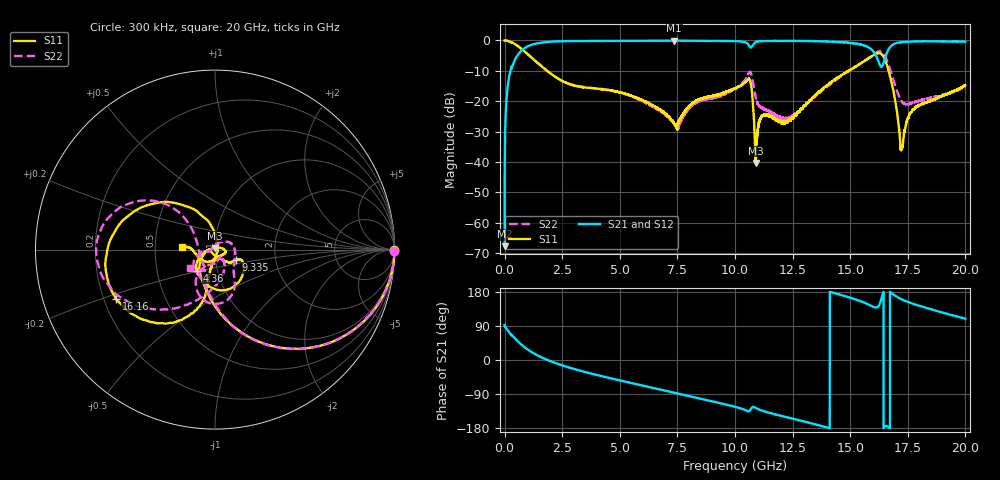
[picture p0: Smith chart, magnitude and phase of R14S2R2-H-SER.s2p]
!{R14S2R2}
!Johanson Technology Inc.
!www.johansontechnology.com
!Test Board Conditions:
!Substrate Type  RO4350B
!Substrate Thickness  20 mil
!Substrate Dk  3.66
!TL Type: GCPW
!TL Trace Width  36 mil
!TL Gap  12 mil
!Electrode orientation  Horizontal
!DUT TOPOLOGY	SERIES
!Mounting Pad LxW  26x36 mil
! Created Wed Nov 25 17:33:21 2020
! 2 Port Network Data from SP1.SP block
! freq  magS11  angS11  magS21  angS21  magS12  angS12  magS22  angS22
# khz S ma R 50
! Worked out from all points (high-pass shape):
!   20001 points, 300 kHz to 20 GHz, reference 50 ohm
!   highest |S21| = -0.06 dB at 7.362 GHz (marker M1); lowest = -67.7 dB at 300 kHz (marker M2)
!   |S21| within 3 dB of the highest: 775.5 MHz to 15.94 GHz (15.16 GHz wide, 181 % of centre); 16.65 GHz to end of sweep
!   lowest |S11| = -40.3 dB at 10.9 GHz (marker M3), VSWR 1.02, Z = 49.9 + j0.954 ohm
!   |S11| at or under -10 dB: 1.845 GHz to 14.93 GHz (13.09 GHz wide, 156 % of centre); 14.93342 GHz to 14.93471 GHz (1.283 MHz wide, 0.00859 % of centre); 16.67 GHz to end of sweep
!   |S22| runs from -29.4 to 0.0 dB; largest |S21 - S12| = 0.016
!   S11 on the Smith chart (normalised r, x): 300 kHz: open; 4.36 GHz: 0.79, -0.19; 9.335 GHz: 1.26, -0.15; 16.16 GHz: 0.25, -0.22; 20 GHz: 0.69, +0.02
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300  0.9984 -0.2  0.0004134 92.1  0.0004495 93.8  0.9979 -0.3
132300  0.983 -11.3  0.1733 78.6  0.1738 78.5  0.9847 -11.3
487300  0.8537 -35.3  0.514 54.3  0.5153 54.4  0.8528 -35.3
1530300  0.3981 -80.9  0.912 9.3  0.9127 9.2  0.3997 -80.1
3334300  0.1716 -119.2  0.9801 -29.1  0.9798 -29.1  0.174 -118.7
4360300  0.155 -131.3  0.983 -44.7  0.9821 -44.7  0.1567 -137.8
6667300  0.07612 -159.8  0.9896 -76.8  0.99 -76.8  0.07216 -169.0
7362300  0.04225 -175.8  0.9935 -86.4  0.9918 -86.4  0.04286 -165.1
9335300  0.1314 -25.5  0.9817 -113.6  0.984 -113.7  0.1221 -24.8
1.00003e7  0.1633 -22.1  0.9727 -123.4  0.9733 -123.4  0.1615 -49.4
1.06323e7  0.2301 -82.2  0.7998 -134.6  0.8028 -134.6  0.3015 -84.6
1.08973e7  0.00963 96.7  0.9343 -126.4  0.9362 -126.5  0.1165 -121.6
1.12353e7  0.05809 -8.9  0.9784 -134.9  0.977 -134.9  0.0755 -89.5
1.21053e7  0.04603 -59.2  0.9836 -148.8  0.9864 -148.8  0.05251 -64.3
1.33343e7  0.111 -103.1  0.9764 -167.5  0.977 -167.4  0.108 -61.0
1.51193e7  0.3501 -106.9  0.8981 162.0  0.9025 161.7  0.3486 -118.1
1.61553e7  0.6164 -153.4  0.5282 138.6  0.5281 139.0  0.6371 -164.3
1.63733e7  0.5892 175.2  0.3706 166.2  0.3681 166.8  0.6443 170.2
1.66673e7  0.3157 127.2  0.7163 -177.3  0.713 -176.4  0.396 138.8
1.72383e7  0.01689 -18.6  0.9392 160.0  0.9399 160.0  0.09902 166.7
1.77793e7  0.07419 -115.4  0.9621 147.3  0.9587 147.1  0.09588 -143.1
2e7  0.1833 175.0  0.9585 108.9  0.9571 109.1  0.1723 -143.0
